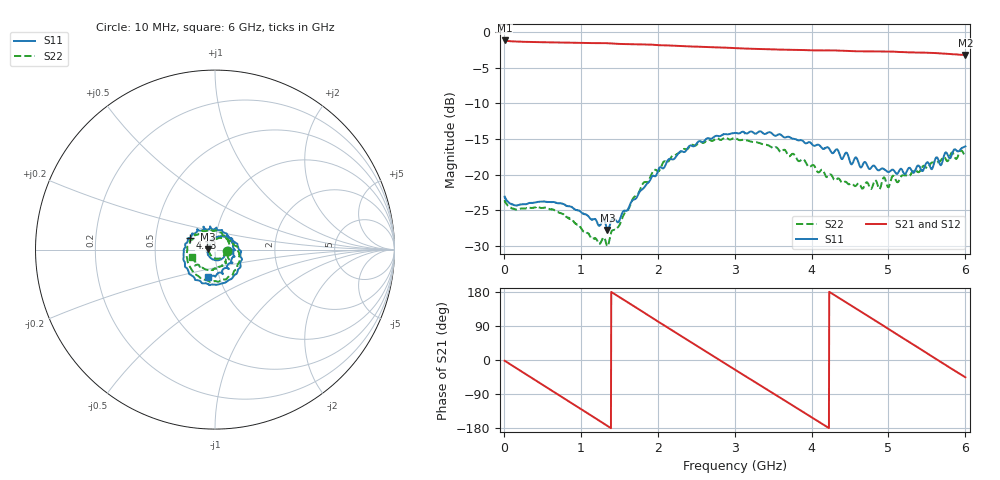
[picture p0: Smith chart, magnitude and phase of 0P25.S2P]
!Agilent Technologies,E5071C,MY46316741,A.11.02
!Date: Thu Jul 30 16:09:20 2020
!Data & Calibration Information:
!Freq	S11:SOLT4(ON)	S21:SOLT4(ON)	S12:SOLT4(ON)	S22:SOLT4(ON)
!PortZ  Port1:50+j0  Port2:50+j0
!Above PortZ is port z conversion or system Z0 setting when saving the data.
!When reading, reference impedance value at option line is always used.
# Hz S dB R 50
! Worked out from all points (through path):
!   1561 points, 10 MHz to 6 GHz, reference 50 ohm
!   highest |S21| = -1.19 dB at 10 MHz (marker M1); lowest = -3.2 dB at 6 GHz (marker M2)
!   group delay of S21, straight-line fit = 354 ps
!   lowest |S11| = -27.8 dB at 1.346 GHz (marker M3), VSWR 1.09, Z = 46.1 + j0.241 ohm
!   |S11| at or under -10 dB: start of sweep to end of sweep
!   |S22| runs from -30.0 to -14.8 dB; largest |S21 - S12| = 0.011
!   S11 on the Smith chart (normalised r, x): 10 MHz: 1.15, -0.02; 4.13 GHz: 0.75, +0.10; 6 GHz: 0.88, -0.27
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1e7  -23.08 -6.7  -1.19 -1.8  -1.19 -1.9  -23.58 -7.8
2.634231e8  -24.13 -19.1  -1.38 -34.5  -1.38 -34.6  -24.73 -20.1
5.475641e8  -23.78 -44.9  -1.44 -71.1  -1.44 -71.2  -24.62 -47.0
7.779487e8  -24.12 -73.1  -1.49 -100.7  -1.48 -100.8  -25.55 -75.6
1.012173e9  -25.34 -110.4  -1.53 -130.8  -1.53 -130.9  -27.62 -116.0
1.346231e9  -27.75 176.3  -1.57 -173.9  -1.57 -174.1  -30.00 152.6
1.649571e9  -23.94 98.3  -1.71 147.3  -1.71 147.0  -24.06 78.2
2.006667e9  -19.35 35.8  -1.84 101.3  -1.84 101.1  -19.52 18.8
2.263929e9  -17.06 -2.3  -1.96 68.4  -1.95 68.0  -17.03 -17.7
2.563429e9  -15.35 -37.3  -2.09 30.5  -2.08 30.1  -15.40 -57.3
2.786135e9  -14.58 -63.0  -2.17 2.3  -2.16 1.8  -14.94 -85.9
3.005e9  -14.14 -87.1  -2.25 -25.6  -2.25 -26.0  -14.83 -114.7
3.266103e9  -14.25 -115.4  -2.37 -58.5  -2.36 -58.9  -15.44 -147.9
3.504167e9  -14.40 -141.1  -2.44 -88.5  -2.43 -89.0  -16.22 179.0
3.742231e9  -14.90 -166.3  -2.49 -118.4  -2.48 -119.0  -17.14 144.5
4.007173e9  -15.75 167.2  -2.56 -151.9  -2.55 -152.6  -18.68 106.9
4.130045e9  -16.19 155.0  -2.58 -167.5  -2.56 -168.1  -19.30 88.7
4.5025e9  -18.27 113.2  -2.68 145.1  -2.68 144.4  -21.29 32.0
4.763603e9  -19.16 78.0  -2.70 112.3  -2.70 111.5  -21.94 -10.2
5.001667e9  -19.60 41.4  -2.73 81.6  -2.73 80.8  -21.78 -40.9
5.516192e9  -18.31 -36.8  -2.90 15.8  -2.90 15.0  -18.98 -102.7
6e9  -16.03 -105.3  -3.22 -45.7  -3.21 -46.6  -17.31 -162.2
